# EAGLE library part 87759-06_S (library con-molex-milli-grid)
HEADER
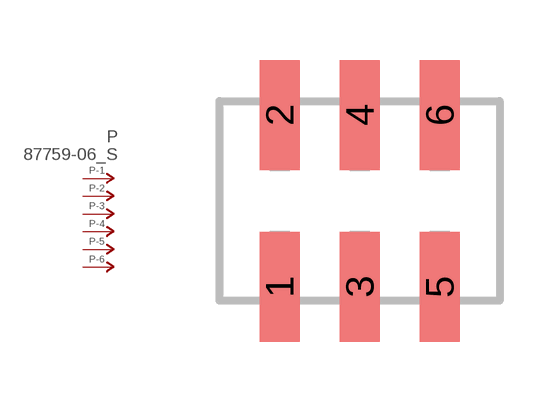
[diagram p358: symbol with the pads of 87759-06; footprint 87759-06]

Designator prefix P; gates -1=P-NV -2=P-N -3=P-N -4=P-N -5=P-N -6=P-N

## 87759-06_S  [87759-06]
1  -1:P  pas
2  -2:P  pas
3  -3:P  pas
4  -4:P  pas
5  -5:P  pas
6  -6:P  pas

## Footprint 87759-06 (pad centres in mm)
HEADER SMD Dual Row, Vertical
smd 1 x 2.75: 1 -2,-2.15; 2 -2,2.15; 3 0,-2.15; 4 0,2.15; 5 2,-2.15; 6 2,2.15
